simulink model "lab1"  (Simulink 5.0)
settings: Solver=ode5  StartTime=0.0  StopTime=50.0  FixedStep=0.01  RelTol=1e-3
libraries: simulink x1

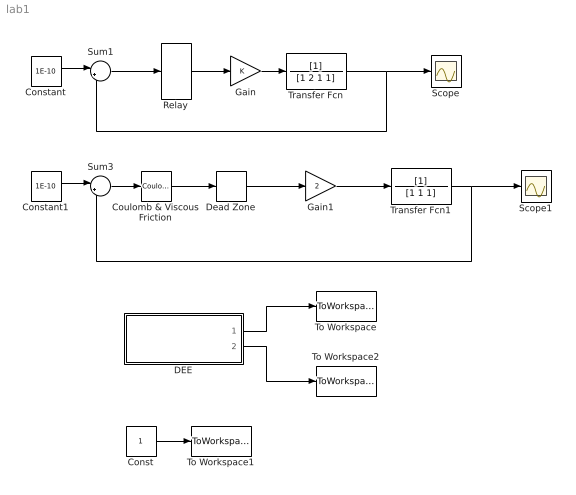
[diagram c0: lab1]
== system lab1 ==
  Const : Constant  ShowAdditionalParam=on  OutDataTypeMode=int8
  Constant : Constant  Value=1E-10  ShowAdditionalParam=on  OutDataTypeMode=double
  Constant1 : Constant  Value=1E-10  ShowAdditionalParam=on  OutDataTypeMode=double
  Coulomb & Viscous Friction : simulink/Discontinuities/Coulomb & Viscous Friction  offset=[1]  gain=0
  DEE : Subsystem
  Dead Zone : DeadZone  LowerValue=-1  UpperValue=1
  Gain : Gain
  Gain1 : Gain  Gain=2
  Relay : Relay  OnSwitchValue=1  OffSwitchValue=-1  OffOutputValue=-1  ShowAdditionalParam=on
  Scope : Scope
  Scope1 : Scope
  Sum1 : Sum  Inputs=|+-
  Sum3 : Sum  Inputs=|+-
  To Workspace : ToWorkspace  VariableName=A_X  SampleTime=-1  SaveFormat=Array
  To Workspace1 : ToWorkspace  VariableName=StartMode  SampleTime=-1  SaveFormat=Array
  To Workspace2 : ToWorkspace  VariableName=A_Y  SampleTime=-1  SaveFormat=Array
  Transfer Fcn : TransferFcn  Denominator=[1 2 1 1]
  Transfer Fcn1 : TransferFcn  Denominator=[1 1 1]
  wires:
  Constant/1 -> Sum1/1
  Transfer Fcn/1 -> Sum1/2, Scope/1
  Constant1/1 -> Sum3/1
  Sum3/1 -> Coulomb & Viscous Friction/1
  Coulomb & Viscous Friction/1 -> Dead Zone/1
  Sum1/1 -> Relay/1
  Relay/1 -> Gain/1
  Gain/1 -> Transfer Fcn/1
  Transfer Fcn1/1 -> Scope1/1, Sum3/2
  Dead Zone/1 -> Gain1/1
  Gain1/1 -> Transfer Fcn1/1
  DEE/1(Port1) -> To Workspace/1
  DEE/2(Port2) -> To Workspace2/1
  Const/1 -> To Workspace1/1

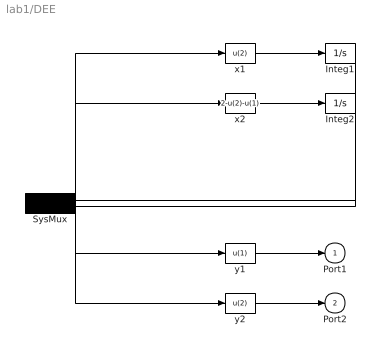
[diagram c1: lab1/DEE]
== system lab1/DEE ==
  Integ1 : Integrator  InitialCondition=-2
  Integ2 : Integrator
  SysMux : Mux  Inputs=2
  x1 : Fcn  Expr=u(2)
  x2 : Fcn  Expr=2-u(2)-u(1)
  y1 : Fcn  Expr=u(1)
  y2 : Fcn  Expr=u(2)
  Port1 : Outport
  Port2 : Outport  Port=2
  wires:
  SysMux/1 -> x1/1, x2/1, y1/1, y2/1
  x1/1 -> Integ1/1
  Integ1/1 -> SysMux/1
  x2/1 -> Integ2/1
  Integ2/1 -> SysMux/2
  y1/1 -> Port1/1
  y2/1 -> Port2/1
